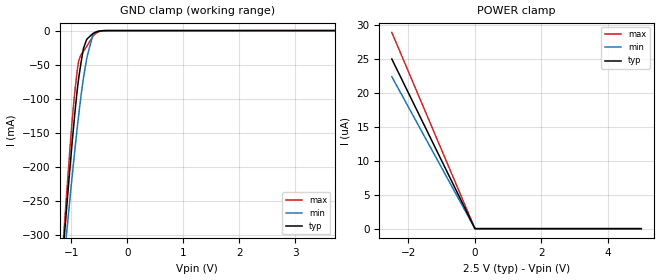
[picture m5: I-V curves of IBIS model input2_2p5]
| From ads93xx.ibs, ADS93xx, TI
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|   input2_2p5 Model
[Model]   input2_2p5
Model_type   Input
Vinl = 0.5
Vinh = 2
|   typ   min   max
C_comp   0.642pF   0.608pF   0.666pF
[Voltage Range]   2.5   2.4   2.6
[Temperature Range]   27   125   -40
[Power Clamp Reference]   2.5   2.4   2.6
[GND Clamp Reference]   0   0   0
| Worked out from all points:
|   GND clamp passes 1 mA (typ) near -0.51 V on its own axis
[GND Clamp]
|   Voltage   I(typ)   I(min)   I(max)
-2.5V     -1.757A    -1.589A    -1.956A
-1.292V   -474.4mA   -480.7mA   -484.6mA
-1.127V   -303.4mA   -334.2mA   -288.9mA
-1.113V   -288.1mA   -321.2mA   -271.5mA
-1.03V    -206.2mA   -250.5mA   -178.4mA
-970mV    -149.7mA   -200.9mA   -117mA
-872.5mV  -72.15mA   -126.2mA   -45.9mA
-782.5mV  -25.84mA   -68.68mA   -29.97mA
-715mV    -11.91mA   -37.04mA   -21.73mA
-617.5mV  -4.497mA   -7.031mA   -8.538mA
-557.5mV  -2.128mA   -1.962mA   -3.922mA
5V        0A         0A         0A
[POWER Clamp]
|   Voltage   I(typ)   I(min)   I(max)
-2.5V     25uA       22.4uA     28.92uA
-2.5mV    19.63nA    17.94nA    23.37nA
12.5mV    0A         0A         0A
5V        0A         0A         0A
